(* Logix 5000 AddOnInstructionDefinition export Banner_S15S_TH_Param_v4; software revision 33.03; part 2 of 2 *)
(* tags used below, declared in another part *)
   S15STH : Banner_S15S_TH_v4;
   Port_Data : Banner_IOL_Port_v4;
   Port : DINT;
   Local_Control : DINT;
   Command_Being_Processed : BOOL;
   Index_Write_Inprocess : INT;
   Inprocess_Index : DINT;
(* Banner_S15S_TH_Param_v4, continued *)

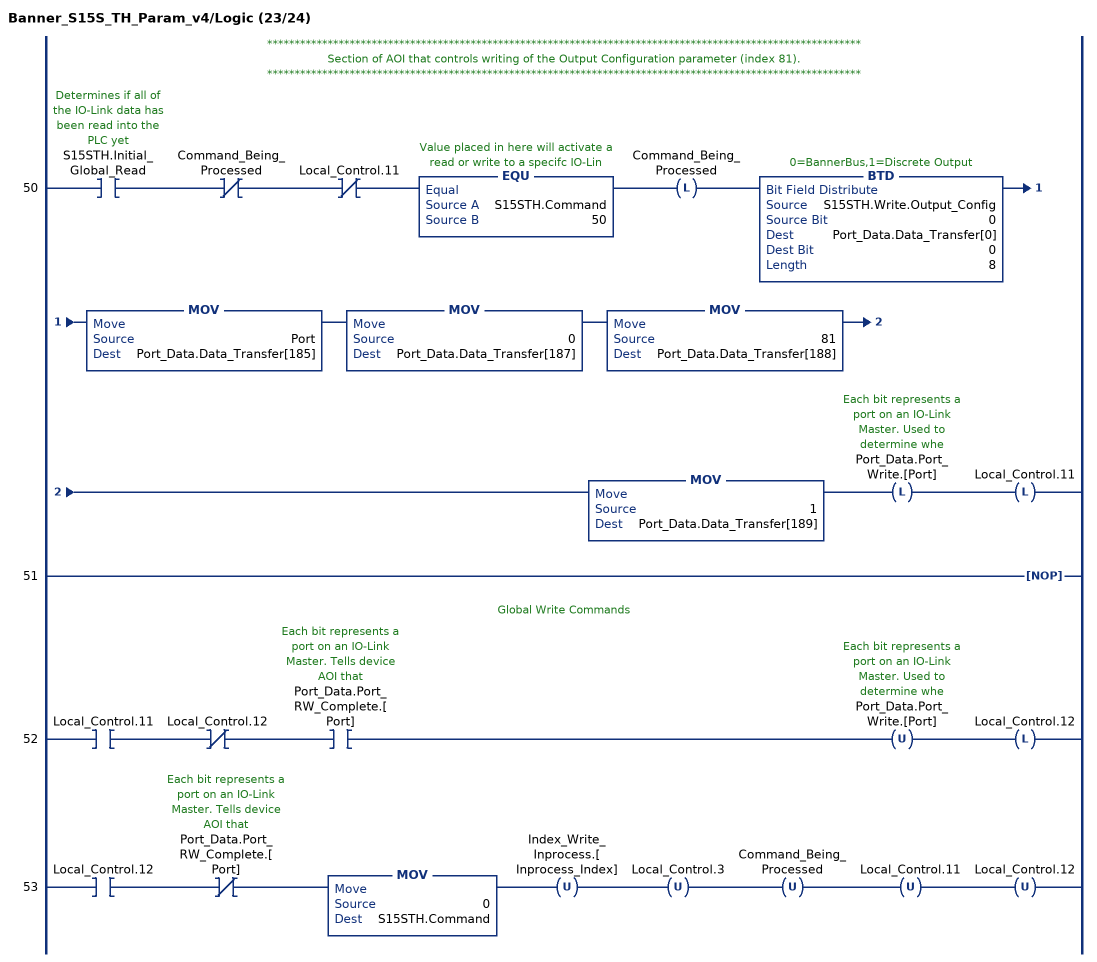
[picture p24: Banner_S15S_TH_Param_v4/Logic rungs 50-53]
   // ************************************************************************************************************
   // Section of AOI that controls writing of the Output Configuration parameter (index 81).
   // ************************************************************************************************************
   50: XIC(S15STH.Initial_Global_Read)XIO(Command_Being_Processed)XIO(Local_Control.11)EQU(S15STH.Command,50)OTL(Command_Being_Processed)BTD(S15STH.Write.Output_Config,0,Port_Data.Data_Transfer[0],0,8)MOV(Port,Port_Data.Data_Transfer[185])MOV(0,Port_Data.Data_Transfer[187])MOV(81,Port_Data.Data_Transfer[188])MOV(1,Port_Data.Data_Transfer[189])OTL(Port_Data.Port_Write.[Port])OTL(Local_Control.11);
   51: NOP();
   // Global Write Commands
   52: XIC(Local_Control.11)XIO(Local_Control.12)XIC(Port_Data.Port_RW_Complete.[Port])OTU(Port_Data.Port_Write.[Port])OTL(Local_Control.12);
   53: XIC(Local_Control.12)XIO(Port_Data.Port_RW_Complete.[Port])MOV(0,S15STH.Command)OTU(Index_Write_Inprocess.[Inprocess_Index])OTU(Local_Control.3)OTU(Command_Being_Processed)OTU(Local_Control.11)OTU(Local_Control.12);
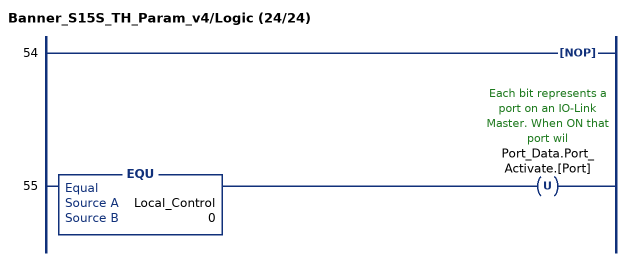
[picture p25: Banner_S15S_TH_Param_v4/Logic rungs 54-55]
   54: NOP();
   55: EQU(Local_Control,0)OTU(Port_Data.Port_Activate.[Port]);
END_ROUTINE
END_ADD_ON_INSTRUCTION
